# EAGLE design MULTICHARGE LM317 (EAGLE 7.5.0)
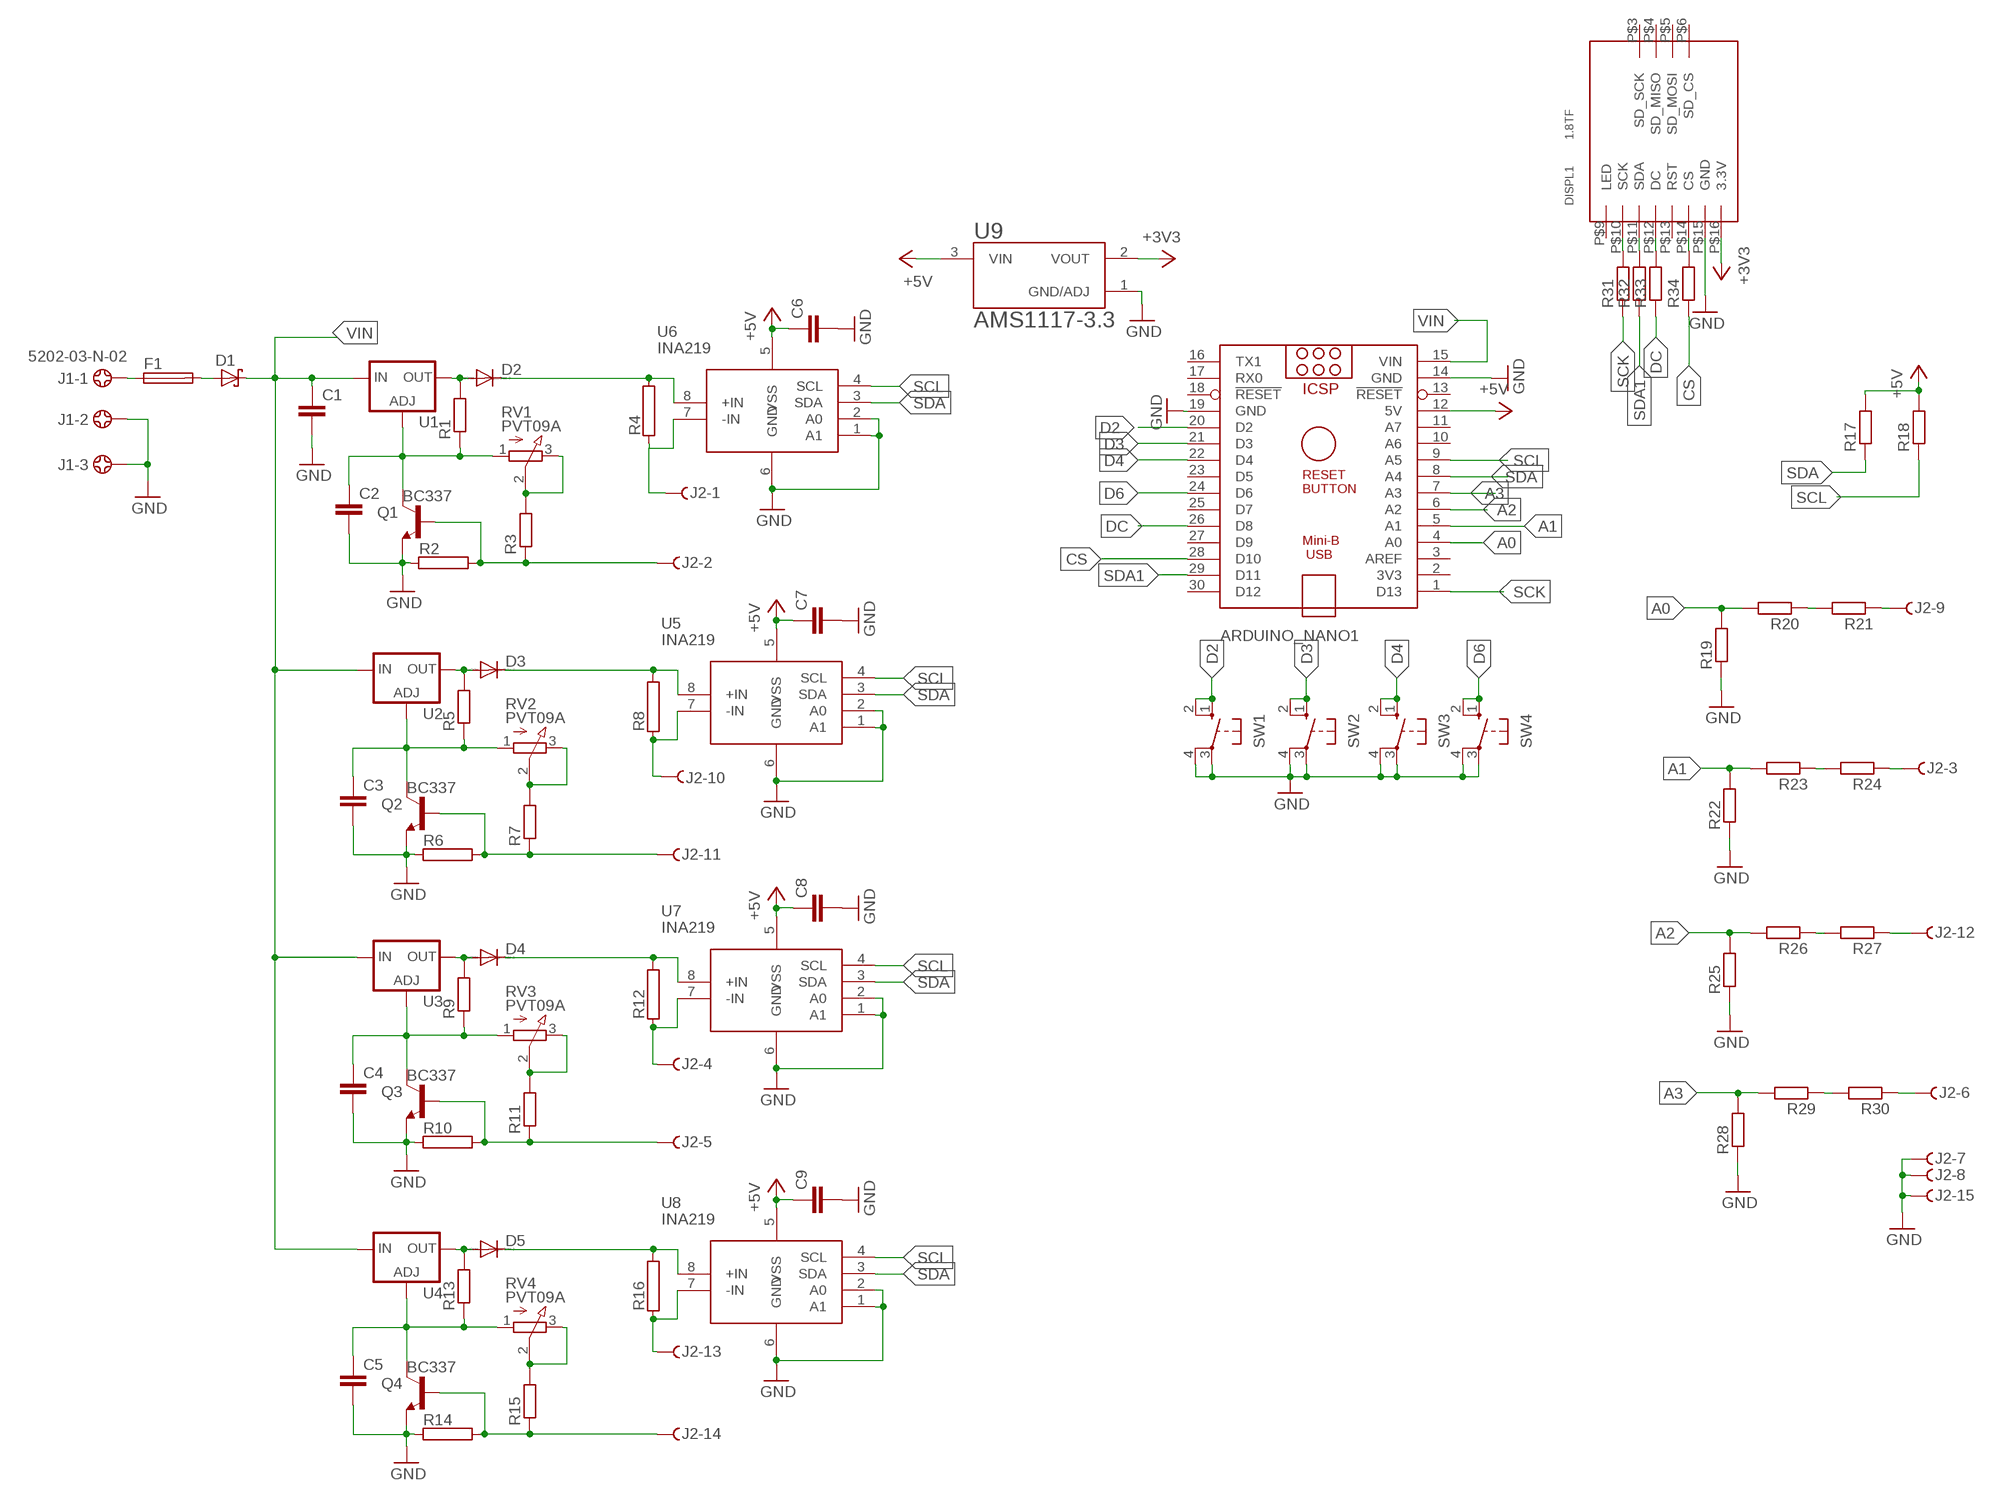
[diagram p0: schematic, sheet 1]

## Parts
ARDUINO_NANO1  ARDUINO_NANO  [ARDUINO_NANO]
C1  C-EUC1206  [C1206]
C2  C-EUC1206  [C1206]
C3  C-EUC1206  [C1206]
C4  C-EUC1206  [C1206]
C5  C-EUC1206  [C1206]
C6  C-EUC0805  [C0805]
C7  C-EUC0805  [C0805]
C8  C-EUC0805  [C0805]
C9  C-EUC1206  [C1206]
D1  MBR1560  [TO220ACS]
D2  CGRM4007-G  [SOD-123_MINI-SMA]
D3  CGRM4007-G  [SOD-123_MINI-SMA]
D4  CGRM4007-G  [SOD-123_MINI-SMA]
D5  CGRM4007-G  [SOD-123_MINI-SMA]
DISPL1  1.8TF  [1.8TFT]
F1  SH22  [SH22]
J1  5202-03-N-02  [5202-03-N-02]
J2  F15.590S  [177-015-212-FEMALE]
Q1  BC337  [TO92]
Q2  BC337  [TO92]
Q3  BC337  [TO92]
Q4  BC337  [TO92]
R1  R-EU_R1206  [R1206]
R2  RAC01  [AC01]
R3  R-EU_R1206  [R1206]
R4  RAC01  [AC01]
R5  R-EU_R1206  [R1206]
R6  RAC01  [AC01]
R7  R-EU_R1206  [R1206]
R8  RAC01  [AC01]
R9  R-EU_R1206  [R1206]
R10  RAC01  [AC01]
R11  R-EU_R1206  [R1206]
R12  RAC01  [AC01]
R13  R-EU_R1206  [R1206]
R14  RAC01  [AC01]
R15  R-EU_R1206  [R1206]
R16  RAC01  [AC01]
R17  R-EU_R1206  [R1206]
R18  R-EU_R1206  [R1206]
R19  R-EU_R1206  [R1206]
R20  R-EU_R1206  [R1206]
R21  R-EU_R1206  [R1206]
R22  R-EU_R1206  [R1206]
R23  R-EU_R1206  [R1206]
R24  R-EU_R1206  [R1206]
R25  R-EU_R1206  [R1206]
R26  R-EU_R1206  [R1206]
R27  R-EU_R1206  [R1206]
R28  R-EU_R1206  [R1206]
R29  R-EU_R1206  [R1206]
R30  R-EU_R1206  [R1206]
R31  R-EU_R1206  [R1206]
R32  R-EU_R1206  [R1206]
R33  R-EU_R1206  [R1206]
R34  R-EU_R1206  [R1206]
RV1  PVT09A  PV09A  [PTV09]
RV2  PVT09A  PV09A  [PTV09]
RV3  PVT09A  PV09A  [PTV09]
RV4  PVT09A  PV09A  [PTV09]
SW1  10-XX  [B3F-10XX]
SW2  10-XX  [B3F-10XX]
SW3  10-XX  [B3F-10XX]
SW4  10-XX  [B3F-10XX]
U1  LM317TS  [317TS]
U2  LM317TS  [317TS]
U3  LM317TS  [317TS]
U4  LM317TS  [317TS]
U5  INA219  [SO08]
U6  INA219  [SO08]
U7  INA219  [SO08]
U8  INA219  [SO08]
U9  AMS1117-3.3  [SOT229P700X180-4N]

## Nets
+3V3: DISPL1.P$16(3.3V) U9.2(VOUT)
+5V: ARDUINO_NANO1.12(5V) C6.1 C7.1 C8.1 C9.1 R17.2 R18.2 U5.5(VSS) U6.5(VSS) U7.5(VSS) U8.5(VSS) U9.3(VIN)
A0: ARDUINO_NANO1.4(A0) R19.2 R20.2
A1: ARDUINO_NANO1.5(A1) R22.2 R23.2
A2: ARDUINO_NANO1.6(A2) R25.2 R26.2
A3: ARDUINO_NANO1.7(A3) R28.2 R29.2
CS: ARDUINO_NANO1.28(D10) R34.1
D2: ARDUINO_NANO1.20(D2) SW1.1(S) SW1.2(S1)
D3: ARDUINO_NANO1.21(D3) SW2.1(S) SW2.2(S1)
D4: ARDUINO_NANO1.22(D4) SW3.1(S) SW3.2(S1)
D6: ARDUINO_NANO1.24(D6) SW4.1(S) SW4.2(S1)
DC: ARDUINO_NANO1.26(D8) R33.1
GND: ARDUINO_NANO1.14(GND) ARDUINO_NANO1.19(GND) C1.2 C2.2 C3.2 C4.2 C5.2 C6.2 C7.2 C8.2 C9.2 DISPL1.P$15(GND) J1.2 J1.3 J2.7 J2.8 J2.15 Q1.1(E) Q2.1(E) Q3.1(E) Q4.1(E) R2.1 R6.1 R10.1 R14.1 R19.1 R22.1 R25.1 R28.1 SW1.3(P) SW1.4(P1) SW2.3(P) SW2.4(P1) SW3.3(P) SW3.4(P1) SW4.3(P) SW4.4(P1) U5.1(A1) U5.2(A0) U5.6(GND) U6.1(A1) U6.2(A0) U6.6(GND) U7.1(A1) U7.2(A0) U7.6(GND) U8.1(A1) U8.2(A0) U8.6(GND) U9.1(GND/ADJ)
N$1: D1.A F1.2
N$2: F1.1 J1.1
N$4: D2.A R1.2 U1.2(OUT)
N$5: C2.1 Q1.3(C) R1.1 RV1.1(A) U1.1(ADJ)
N$6: R3.2 RV1.2(S) RV1.3(E)
N$7: R23.1 R24.2
N$8: J2.2 Q1.2(B) R2.2 R3.1
N$9: D3.A R5.2 U2.2(OUT)
N$10: C3.1 Q2.3(C) R5.1 RV2.1(A) U2.1(ADJ)
N$11: J2.11 Q2.2(B) R6.2 R7.1
N$12: D2.C R4.2 U6.8(+IN)
N$13: J2.1 R4.1 U6.7(-IN)
N$14: R7.2 RV2.2(S) RV2.3(E)
N$15: D3.C R8.2 U5.8(+IN)
N$16: J2.10 R8.1 U5.7(-IN)
N$17: D4.A R9.2 U3.2(OUT)
N$18: C4.1 Q3.3(C) R9.1 RV3.1(A) U3.1(ADJ)
N$19: J2.5 Q3.2(B) R10.2 R11.1
N$20: R11.2 RV3.2(S) RV3.3(E)
N$21: D4.C R12.2 U7.8(+IN)
N$22: J2.4 R12.1 U7.7(-IN)
N$23: D5.A R13.2 U4.2(OUT)
N$24: C5.1 Q4.3(C) R13.1 RV4.1(A) U4.1(ADJ)
N$25: J2.14 Q4.2(B) R14.2 R15.1
N$26: R15.2 RV4.2(S) RV4.3(E)
N$27: D5.C R16.2 U8.8(+IN)
N$28: J2.13 R16.1 U8.7(-IN)
N$29: R20.1 R21.2
N$30: J2.9 R21.1
N$31: J2.3 R24.1
N$32: R26.1 R27.2
N$34: R29.1 R30.2
N$35: J2.12 R27.1
N$37: J2.6 R30.1
N$50: DISPL1.P$10(SCK) R31.2
N$51: DISPL1.P$11(SDA) R32.2
N$52: DISPL1.P$12(DC) R33.2
N$53: DISPL1.P$14(CS) R34.2
SCK: ARDUINO_NANO1.1(D13) R31.1
SCL: ARDUINO_NANO1.9(A5) R18.1 U5.4(SCL) U6.4(SCL) U7.4(SCL) U8.4(SCL)
SDA: ARDUINO_NANO1.8(A4) R17.1 U5.3(SDA) U6.3(SDA) U7.3(SDA) U8.3(SDA)
SDA1: ARDUINO_NANO1.29(D11) R32.1
VIN: ARDUINO_NANO1.15(VIN) C1.1 D1.C U1.3(IN) U2.3(IN) U3.3(IN) U4.3(IN)
Unconnected: ARDUINO_NANO1.2(3V3) ARDUINO_NANO1.3(AREF) ARDUINO_NANO1.10(A6) ARDUINO_NANO1.11(A7) ARDUINO_NANO1.13(!RESET) ARDUINO_NANO1.16(TX1) ARDUINO_NANO1.17(RX0) ARDUINO_NANO1.18(!RESET) ARDUINO_NANO1.23(D5) ARDUINO_NANO1.25(D7) ARDUINO_NANO1.27(D9) ARDUINO_NANO1.30(D12) DISPL1.P$3(SD_SCK) DISPL1.P$4(SD_MISO) DISPL1.P$5(SD_MOSI) DISPL1.P$6(SD_CS) DISPL1.P$9(LED) DISPL1.P$13(RST)

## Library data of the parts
ARDUINO_NANO1 = ArduinoNanoV30:ARDUINO_NANO: Arduino Nano V3.0 Overview: The Arduino Nano is a small, complete, and breadboard-friendly board based on the ATmega328 (Arduino Nano 3.x) or ATmega168 (Arduino Nano 2.x). It has more or less the same functionality of the Arduino Duemilanove, but in a different package. It lacks only a DC power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
C1-C9 = rcl:C-EU: CAPACITOR, European symbol
D1 = diode:MBR1560
D2-D5 = diode:CGRM400*-G: Molded plasitc,JEDEC SOD-123/Mini SMA
DISPL1 = tft_1_8_1_44_oled_0_96:1.8TF
F1 = fuse:SH22: FUSE HOLDER; OC_FARNELL: unknown; OC_NEWARK: unknown
J1 = con-ebyelectro:5202-03-N-02: Barrier Blocks Sreies 5202 Source: http://www.ebyelectro.com/PDF/5202-XX-N-02.pdf; OC_FARNELL: unknown; OC_NEWARK: unknown
J2 = con-subd:F15?S: SUB-D; OC_FARNELL: unknown; OC_NEWARK: unknown
Q1-Q4 = transistor:BC337: NPN TRANSISTOR
R1 R3 R5 R7 R9 R11 R13 R15 R17-R34 = rcl:R-EU_: RESISTOR, European symbol
R2 R4 R6 R8 R10 R12 R14 R16 = resistor-power:R: Power Resitor; OC_FARNELL: unknown; OC_NEWARK: unknown
RV1-RV4 = pot:PV09A
SW1-SW4 = switch-omron:10-XX: OMRON SWITCH; MPN: B3F-1000; OC_FARNELL: 176432; OC_NEWARK: 36M3542
U1-U4 = v-reg:LM317TS: VOLTAGE REGULATOR
U5-U8 = burr-brown:INA219: Bidirectional Current/Power Monitor With I2C Interface
U9 = AMS1117-3.3:AMS1117-3.3: Check availability; AVAILABILITY: Not in stock; CHECK_PRICES: https://www.snapeda.com/parts/AMS1117-3.3/Advanced+Monolithic+Systems/view-part/?ref=eda; DESCRIPTION: Sot223/Pkg 1-Amp 3.3-Volt Low Drop Out Voltage Regulatator; MF: Advanced Monolithic Systems; MP: AMS1117-3.3; PACKAGE: SOT-223 Seeed Technology; PRICE: None; SNAPEDA_LINK: https://www.snapeda.com/parts/AMS1117-3.3/Advanced+Monolithic+Systems/view-part/?ref=snap

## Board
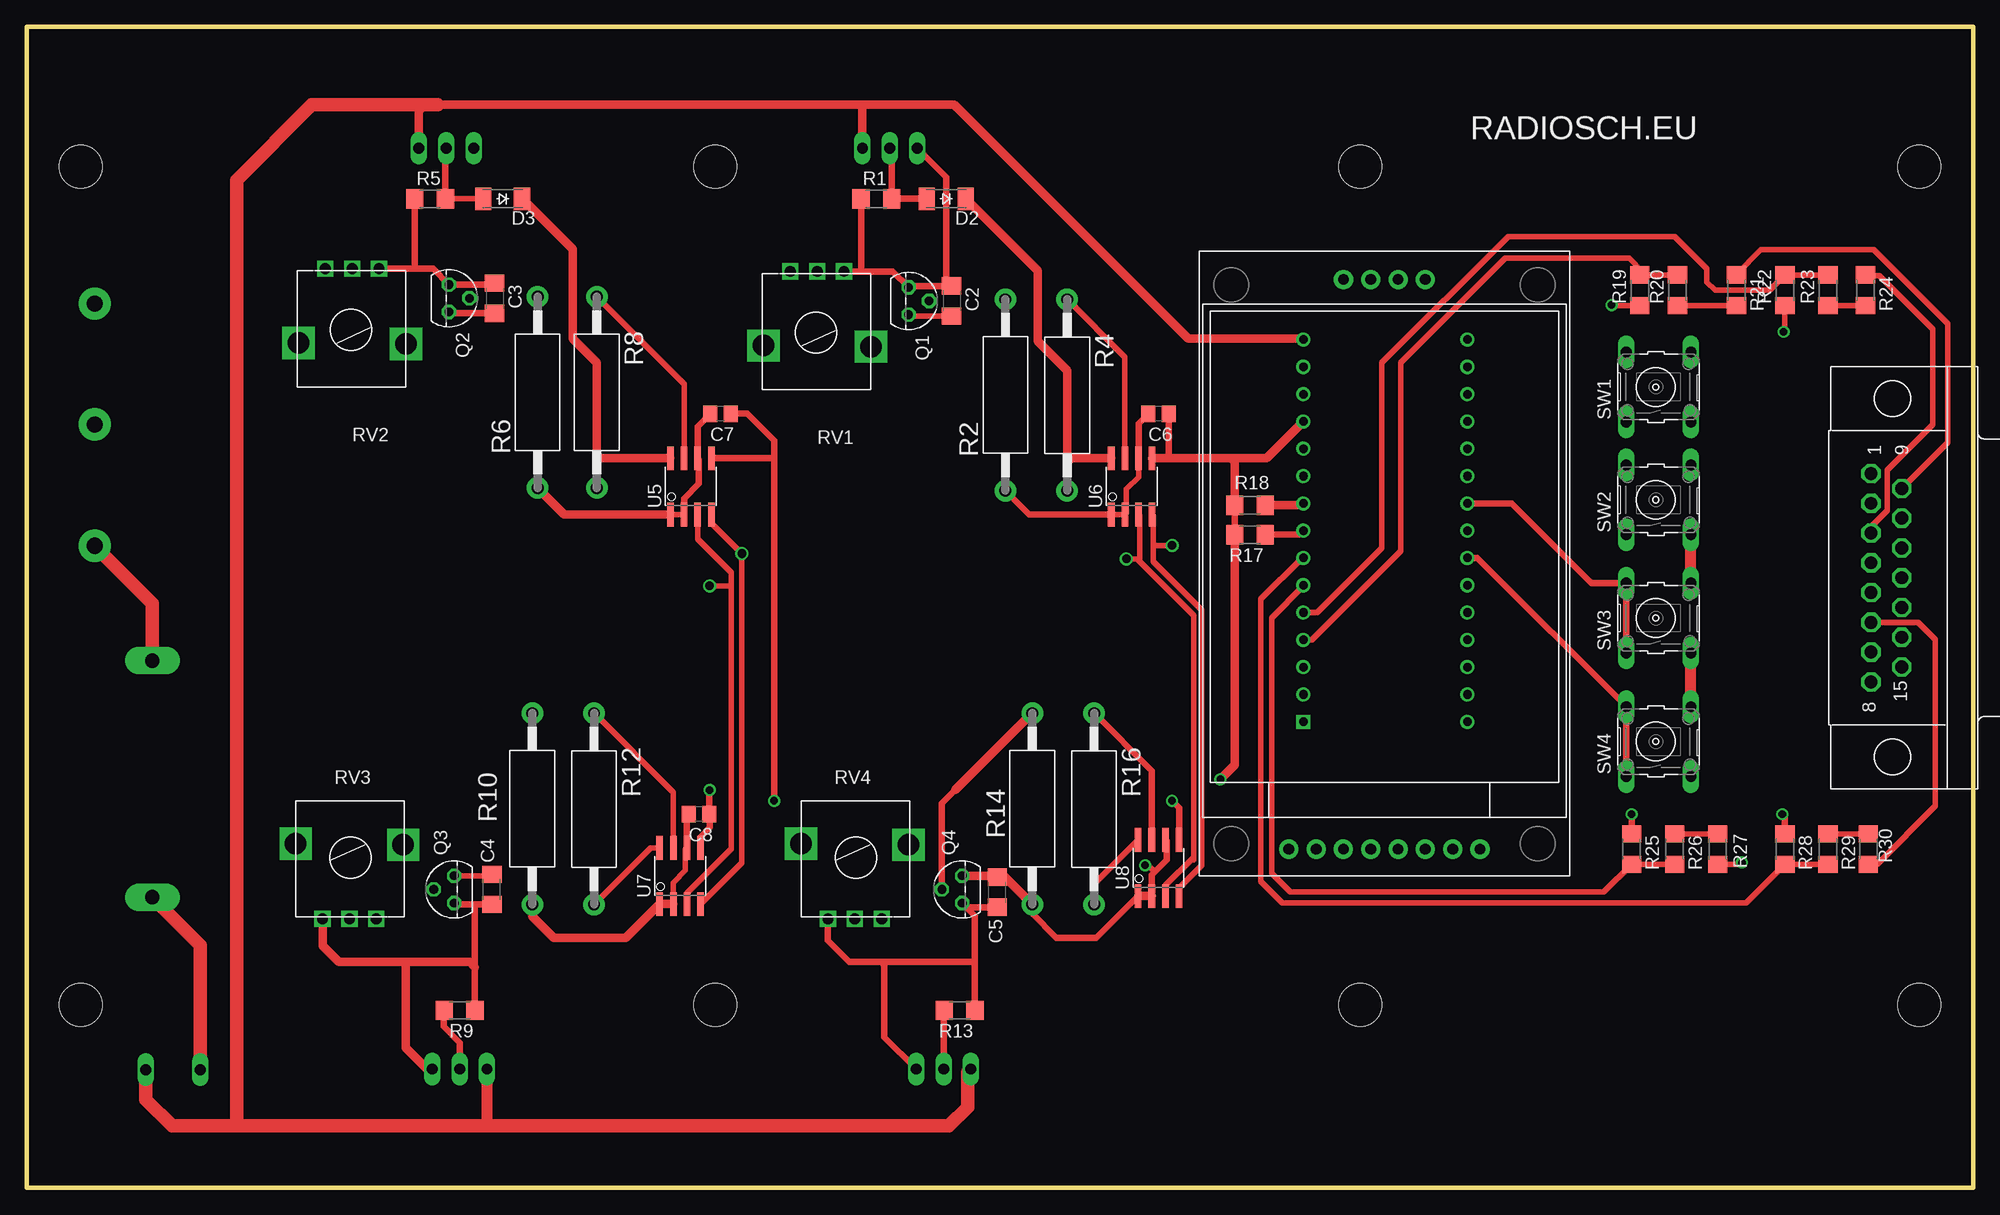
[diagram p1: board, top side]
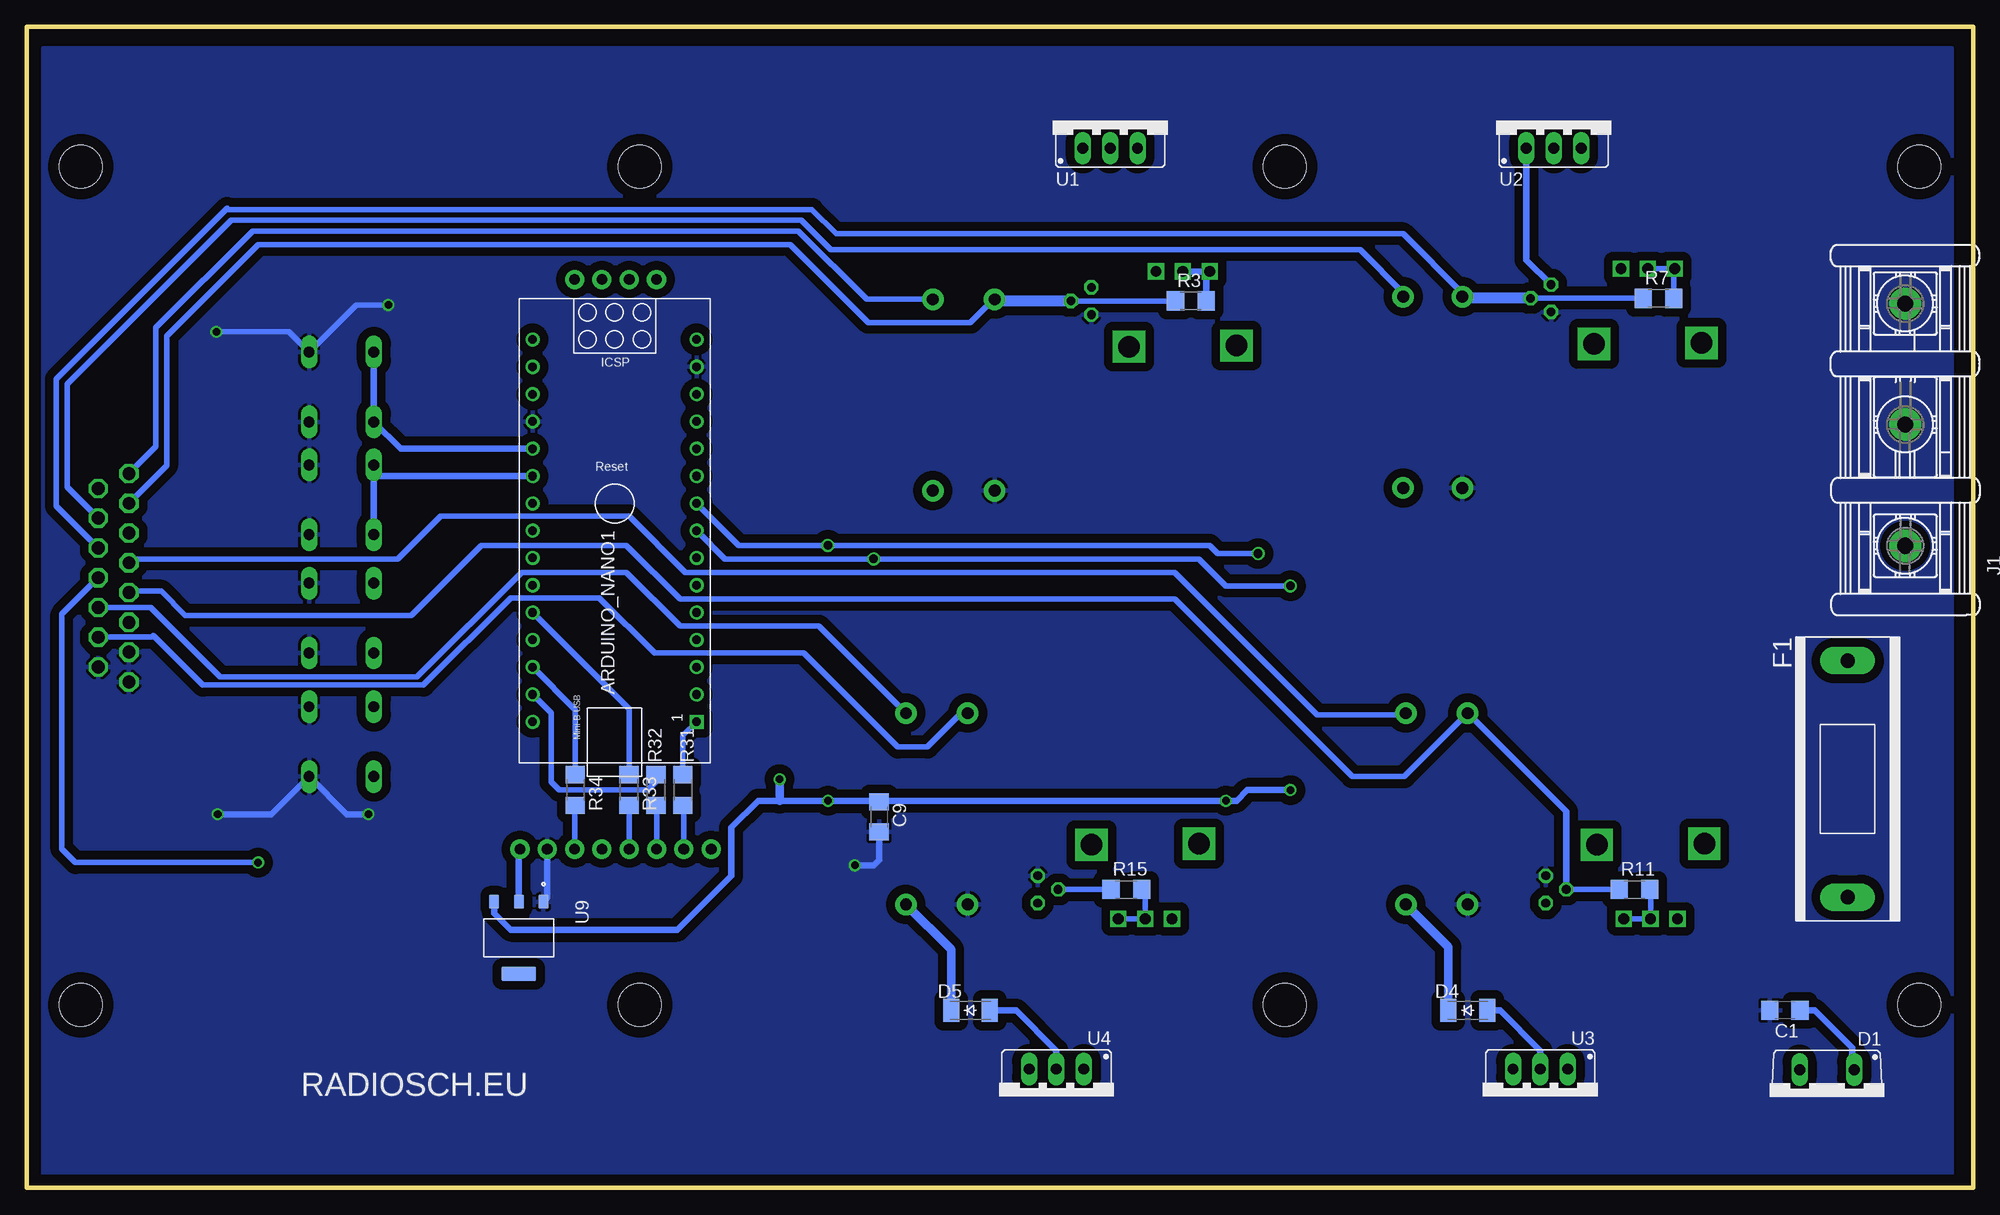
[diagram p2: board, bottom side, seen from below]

Size 181 x 108 mm. Coordinates in mm from the lower left corner, seen from the top.
Outline: 0,0 181,0 181,108 0,108 0,0
Copper layers (1*16): Top 0.035mm / dielectric 1.5mm / Bottom 0.035mm
Design rules "default": minimum track width 10mil, minimum drill 24mil, track to track 8mil, track to pad 8mil, pad to pad 8mil, via to via 8mil, smd to smd 8mil, copper to edge 40mil, drill to drill 8mil, minimum pad ring 10mil, minimum via ring 8mil, stop-mask expansion 4mil, vias tented up to drill 0mil, thermal gap 10mil
Holes 4 mm at 5,95 5,17 176,17 176,95 64,17 124,17 64,95 124,95

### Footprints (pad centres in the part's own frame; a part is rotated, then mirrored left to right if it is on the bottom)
ARDUINO_NANO = drill 0.8 square: 1 -20.32,-7.62 | drill 0.8: 2 -17.78,-7.62; 3 -15.24,-7.62; 4 -12.7,-7.62; 5 -10.16,-7.62; 6 -7.62,-7.62; 7 -5.08,-7.62; 8 -2.54,-7.62; 9 0,-7.62; 10 2.54,-7.62; 11 5.08,-7.62; 12 7.62,-7.62; 13 10.16,-7.62; 14 12.7,-7.62; 15 15.24,-7.62; 16 15.24,7.62; 17 12.7,7.62; 18 10.16,7.62; 19 7.62,7.62; 20 5.08,7.62; 21 2.54,7.62; 22 0,7.62; 23 -2.54,7.62; 24 -5.08,7.62; 25 -7.62,7.62; 26 -10.16,7.62; 27 -12.7,7.62; 28 -15.24,7.62; 29 -17.78,7.62; 30 -20.32,7.62
C1206 = smd 1.6 x 1.8: 1 -1.4,0; 2 1.4,0
C0805 = smd 1.3 x 1.5: 1 -0.95,0; 2 0.95,0
TO220ACS = drill 1.016 long: A 2.54,-2.54; C -2.54,-2.54
SOD-123_MINI-SMA = smd 1.5 x 2.1: A 1.8,0; C -1.8,0
1.8TFT = drill 1 pad 1.778: P$3 55.5,21.05; P$4 55.5,18.52; P$5 55.5,15.98; P$6 55.5,13.44; P$9 2.5,26.14; P$10 2.5,23.6; P$11 2.5,21.06; P$12 2.5,18.52; P$13 2.5,15.98; P$14 2.5,13.44; P$15 2.5,10.9; P$16 2.5,8.36
SH22 = drill 1.321 pad 2.54 long: 1 -10.998,0; 2 10.998,0
5202-03-N-02 = drill 1.5 pad 3: 1 -9.29,0; 2 2,0; 3 13.25,0
177-015-212-FEMALE = drill 1.194 pad 1.524 octagon: 1 -9.69,-1.99; 2 -6.921,-1.99; 3 -4.153,-1.99; 4 -1.384,-1.99; 5 1.384,-1.99; 6 4.153,-1.99; 7 6.921,-1.99; 8 9.69,-1.99; 9 -8.306,0.854; 10 -5.537,0.854; 11 -2.769,0.854; 12 0,0.854; 13 2.769,0.854; 14 5.537,0.854; 15 8.306,0.854
TO92 = drill 0.813 octagon: 1 1.27,0; 2 0,1.905; 3 -1.27,0
R1206 = smd 1.6 x 1.803: 1 -1.422,0; 2 1.422,0
AC01 = drill 1.1 pad 2: 1 -8.9,0; 2 8.9,0
PTV09 = drill 1 square: 1 -2.5,0; 2 0,0; 3 2.5,0 | drill 2 square: P$4 -5,7; P$5 5,6.9
B3F-10XX = drill 1.016 long: 1 -3.251,2.761; 2 3.251,2.761; 3 -3.251,-3.261; 4 3.251,-3.261
317TS = drill 1.016 long: 1 -2.54,-2.54; 2 0,-2.54; 3 2.54,-2.54
SO08 = smd 0.61 x 2.21: 1 -1.905,-2.616; 2 -0.635,-2.616; 3 0.635,-2.616; 4 1.905,-2.616; 5 1.905,2.616; 6 0.635,2.616; 7 -0.635,2.616; 8 -1.905,2.616
SOT229P700X180-4N = smd 1.31 x 0.93: 1 -3.345,2.29; 2 -3.345,0; 3 -3.345,-2.29 | smd 1.31 x 3.24: 4 3.345,0

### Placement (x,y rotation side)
ARDUINO_NANO1  126.34,63.67 90 bottom
C1  17.5,16.5 180 bottom
C2  86,82.5 270 top
C3  43.5,82.75 270 top
C4  43.25,27.75 90 top
C5  90.25,27.5 90 top
C6  105.25,72 180 top
C7  64.5,72 180 top
C8  62.5,34.75 180 top
C9  101.75,34.5 270 bottom
D1  13.6,8.44 180 bottom
D2  85.5,92 180 top
D3  44.25,92 180 top
D4  47,16.5 0 bottom
D5  93.25,16.5 0 bottom
DISPL1  143.5,29 90 top
F1  11.67,38.03 270 bottom
J1  6.32,69.01 90 bottom
J2  173.5,56.75 270 top
Q1  82,82.5 270 top
Q2  39.25,82.75 270 top
Q3  39.75,27.75 90 top
Q4  87,27.75 90 top
R1  79,92 0 top
R2  91,73.75 90 top
R3  72.75,82.5 0 bottom
R4  96.75,73.75 270 top
R5  37.5,92 0 top
R6  47.5,74 90 top
R7  29.25,82.75 0 bottom
R8  53,74 270 top
R9  40.25,16.5 180 top
R10  47,35.25 90 top
R11  31.5,27.75 0 bottom
R12  52.75,35.25 270 top
R13  86.75,16.5 180 top
R14  93.5,35.25 90 top
R15  78.75,27.75 0 bottom
R16  99.25,35.25 270 top
R17  113.75,60.75 180 top
R18  113.75,63.5 180 top
R19  150,83.5 90 top
R20  153.5,83.5 90 top
R21  159,83.5 270 top
R22  163.5,83.5 90 top
R23  167.5,83.5 90 top
R24  171,83.5 270 top
R25  149.25,31.5 270 top
R26  153.25,31.5 270 top
R27  157.25,31.5 90 top
R28  163.5,31.5 270 top
R29  167.5,31.5 270 top
R30  171.25,31.5 90 top
R31  120,37 270 bottom
R32  122.5,37 270 bottom
R33  125,37 270 bottom
R34  130,37 270 bottom
RV1  73.5,85.25 180 top
RV2  30.25,85.5 180 top
RV3  30,25 0 top
RV4  77,25 0 top
SW1  151.5,74.5 90 top
SW2  151.5,64 90 top
SW3  151.5,53 90 top
SW4  151.5,41.5 90 top
U1  80.25,99.25 0 bottom
U2  39,99.25 0 bottom
U3  40.25,8.5 180 bottom
U4  85.25,8.5 180 bottom
U5  61.75,65.25 0 top
U6  102.75,65.25 0 top
U7  60.75,29 0 top
U8  105.25,29.75 0 top
U9  135.25,23.25 270 bottom

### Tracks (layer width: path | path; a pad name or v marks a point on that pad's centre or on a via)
+3V3
  Bottom 0.61: U9.2 135.25,31.39 DISPL1.P$16
+5V  (via drill 0.7)
  Top 0.61: U8.5 107.16,35.34 v106.5,36 | R18.2 R17.2 | U7.5 62.66,32.66 63.5,33.5 63.5,34.7 C8.1 63.45,36.95 v63.5,37 | 69.5,68 69.5,69.5 67,72 C7.1 | 69.5,68 v69.5,36 | U5.5 69.37,67.87 69.5,68 | C6.1 106.2,67.94 106.12,67.87
  Top 0.813: 104.66,67.84 U6.5 106.12,67.87 112,67.87 | 112,67.87 115.3,67.87 ARDUINO_NANO1.12 | R18.2 112.33,67.54 112,67.87 | R17.2 112.33,39.33 v111,38
  Bottom 0.61: U9.3 137.54,25.54 136,24 120.5,24 115.5,29 115.5,33.5 113,36 111,36 v106.5,36 101.85,36 C9.1 101.65,36 v69.5,36 68.5,36 67.5,37 v63.5,37
  Bottom 0.813: v111,38 111,36
A0
  Top 0.5: 150.25,85.25 149,86.5 137.5,86.5 127.75,76.75 127.75,59.25 119.47,50.97 ARDUINO_NANO1.4 | 150.25,85.25 150.58,84.92 R20.2 | R19.2 150,85 150.25,85.25
A1
  Top 0.5: R23.2 R22.2 162.08,83.5 157,83.5 156.25,84.25 156.25,85.5 153.25,88.5 137.75,88.5 126,76.75 126,59.5 120.01,53.51 ARDUINO_NANO1.5
A2
  Top 0.5: ARDUINO_NANO1.6 118.72,55.97 115.75,53 115.75,29.25 117.5,27.5 146.67,27.5 R25.2 R26.2
A3
  Top 0.5: ARDUINO_NANO1.7 118.59,58.59 114.75,54.75 114.75,28.5 116.75,26.5 159.92,26.5 R28.2 R29.2
CS
  Bottom 0.5: R34.1 130,44.47 ARDUINO_NANO1.28
D2
  Bottom 0.61: SW1.2 SW1.1 146.24,68.75 ARDUINO_NANO1.20
D3
  Bottom 0.61: SW2.1 148.74,66.75 | 148.74,66.75 SW2.2 | ARDUINO_NANO1.21 148.2,66.21 148.74,66.75
D4
  Top 0.61: SW3.1 SW3.2 145.5,56.25 138.08,63.67 ARDUINO_NANO1.22
D6
  Top 0.61: ARDUINO_NANO1.24 134.9,58.59 SW4.2 SW4.1
DC
  Bottom 0.5: R33.1 125,44.55 ARDUINO_NANO1.26
GND  (via drill 0.7)
  Top 0.5: U5.2 U5.1 | U7.2 60.12,28.36 61.25,29.5 61.25,31.48 U7.6 | Q3.1 43.12,29.02 C4.2 | 47,25.25 R10.1 | R19.1 147.42,82.08 v147.38,82.12 | R22.1 163.5,79.75 v163.38,79.62 | U6.6 103.39,66.14 102.25,65 102.25,62.77 U6.2 U6.1 | C2.2 82.13,81.1 Q1.1
  Top 0.61: R14.1 93.5,25.5 95.75,23.25 99.46,23.25 U8.1 | U8.2 104.61,29.11 104.88,29.38 | 104.88,29.38 106,30.5 106,32.25 U8.6 | C5.2 90.25,29.02 | v104,30 104.25,30 104.88,29.38 | C3.2 39.38,81.35 Q2.1 | U7.6 61.38,34.59 C8.2 | U5.2 61.12,64.11 62.5,65.5 62.5,67.75 U5.6 62.38,70.83 C7.2 | R25.1 v149.25,34.75 | R28.1 163.5,34.5 v163.25,34.75 | U6.1 93.22,62.63 R2.1 | U6.6 103.39,71.08 C6.2
  Top 0.813: 47,25.25 49,23.25 55.71,23.25 U7.1 U7.2 | Q4.1 90.25,29.02 90.83,29.02 R14.1 | U8.1 U8.2 | U5.1 49.97,62.63 R6.1
  Top 1.016: SW4.4 SW3.3 | SW3.4 SW2.3
  Bottom 0.5: v147.38,82.12 150.39,82.12 SW1.4 156.63,79.62 v163.38,79.62
  Bottom 0.61: DISPL1.P$15 132.6,26.95 U9.1 | C9.2 101.75,30.5 102.25,30 v104,30 | v149.25,34.75 151.26,34.75 SW4.3 158.26,34.75 v163.25,34.75
  Bottom 0.813: 46.87,26.48 R10.1
  pour Bottom (isolate 0.813): 2,106 179.5,106 179.5,1 2,1
N$1
  Top 1.27: D1.A 16.14,22.56 F1.2
N$2
  Top 1.27: F1.1 11.67,54.37 J1.1
N$4
  Top 0.61: D2.A R1.2 80.42,96.54 U1.2
N$5
  Top 0.61: RV1.1 77.5,85.25 | 77.5,85.25 80.52,85.25 Q1.3 82.13,83.9 C2.1 85.5,84.4 85.5,94 U1.1 | R1.1 77.58,85.33 77.5,85.25
N$6
  Bottom 0.61: R3.2 71.33,84.92 RV1.3 RV1.2
N$7
  Top 0.5: R23.1 R24.2
N$8
  Bottom 0.5: R2.2 91.1,82.65 93.25,80.5 102.75,80.5 110,87.75 159.5,87.75 168,79.25 168,67.18 J2.2 | R3.1 Q1.2
  Bottom 1.016: Q1.2 90.85,82.5 R2.2
N$9
  Top 0.5: R5.2 D3.A
  Top 0.61: R5.2 38.92,96.88 U2.2
N$10
  Top 0.61: RV2.1 36,85.5 | 36,85.5 37.77,85.5 Q2.3 39.98,84.02 40,84 43.35,84 C3.1 | R5.1 36.08,85.58 36,85.5
  Bottom 0.61: U2.1 41.54,86.31 Q2.3
N$11
  Bottom 0.5: R6.2 47.5,83.25 53,88.75 105.75,88.75 108,91 162.25,91 162.38,91.12 178.25,75.25 178.25,63.41 J2.11 | R7.1 Q2.2
  Bottom 1.016: Q2.2 47.35,82.75 R6.2
N$12
  Top 0.813: D2.C 94,85.3 94,78.75 96.75,76 96.75,67.5 | R4.2 96.75,67.5 | U6.8 97.12,67.87 96.75,67.5
N$13
  Top 0.5: U6.7 102.11,77.28 R4.1
  Bottom 0.5: J2.1 169,68.95 169,80 160,89 109.25,89 102.9,82.65 R4.1
N$14
  Bottom 0.5: R7.2 27.83,85.42 RV2.3 RV2.2
N$15
  Top 0.813: R8.2 53,67.75 | 53,67.75 53,76.75 50.75,79 50.75,87.3 D3.C | U5.8 53.12,67.87 53,67.75
N$16
  Top 0.5: U5.7 61.12,74.78 R8.1
  Bottom 0.5: R8.1 53,83.25 57,87.25 106.25,87.25 109,90 162,90 177.25,74.75 177.25,65.18 J2.10
N$17
  Top 0.61: 38.75,16.42 38.75,15 40.25,13.5 U3.2
  Top 0.813: 38.75,16.42 R9.2
  Bottom 0.61: D4.A 44,16.5 40.25,12.75 U3.2
N$18
  Top 0.61: C4.1 41.75,26.35 | 41.75,26.35 39.88,26.35 Q3.3 | R9.1 41.67,20.5 41.67,26.27 41.75,26.35
  Top 0.813: RV3.1 27.5,22.5 29,21 35,21 | 35,21 41.17,21 41.67,20.5 | U3.1 37.21,11.04 35.25,13 35.25,20.75 35,21
N$19
  Bottom 0.5: Q3.2 R11.1 | J2.5 171.38,55.5 168.5,55.5 166.25,53.25 145.25,53.25 138.75,59.75 125.25,59.75 120.25,54.75 74.25,54.75 57.75,38.25 52.9,38.25 R10.2
  Bottom 0.61: Q3.2 37.84,34.99 R10.2
  Bottom 0.813: R10.2 47.35,44.15
N$20
  Bottom 0.5: R11.2 30,27.67 RV3.2 RV3.3
N$21
  Top 0.5: U7.8 58.02,31.62 R12.2
  Bottom 0.813: D4.C 48.8,22.4 R12.2
N$22
  Top 0.5: U7.7 60.12,36.78 R12.1
  Bottom 0.5: J2.4 171.14,58.5 146.5,58.5 142.5,62.5 125,62.5 119.75,57.25 74.25,57.25 61,44 52.9,44 R12.1
N$23
  Top 0.61: U4.2 85.25,16.42 R13.2
  Bottom 0.61: D5.A 89,16.5 85.25,12.75 U4.2
N$24
  Top 0.61: R13.1 88.17,21 | 88.17,21 88.17,25.31 Q4.3 87.38,26.1 C5.1 | RV4.1 74.5,23 76.5,21 79.5,21 | 79.5,21 88.17,21 | U4.1 79.75,14 79.75,20.75 79.5,21
N$25
  Top 0.61: Q4.2 85.09,35.74 86.34,36.99
  Top 0.813: 86.34,36.99 R14.2
  Bottom 0.5: Q4.2 R15.1 | R14.2 94.1,44.15 97.25,41 100,41 108.75,49.75 122.62,49.75 127.75,54.88 136,54.88 144.12,46.75 164.62,46.75 168.81,50.94 169.09,51.21 | 169.09,51.21 169.25,51.38 | J2.14 169.09,51.21
N$26
  Bottom 0.5: R15.2 77,27.42 RV4.2 RV4.3
N$27
  Top 0.5: R16.2 99.25,28.27 U8.8
  Bottom 0.813: D5.C 95.05,22.15 R16.2
N$28
  Top 0.61: U8.7 104.61,38.78 R16.1
  Bottom 0.5: J2.13 169.48,53.98 163,47.5 144.75,47.5 135,57.25 125.25,57.25 120.25,52.25 107.35,52.25 R16.1
N$29
  Top 0.5: R20.1 R21.2
N$30
  Top 0.5: J2.9 178.62,69.33 178.62,80.38 171.75,87.25 161.25,87.25 159,85 R21.1
N$31
  Top 0.5: J2.3 171.51,61.51 173,63 173,66.75 177.25,71 177.25,79.88 172.25,84.88 171.05,84.88 R24.1
N$32
  Top 0.5: R27.2 R26.1
N$34
  Top 0.5: R29.1 R30.2
N$35  (via drill 0.7)
  Top 0.5: R27.1 159.33,30.08 v159.5,30.25
  Bottom 0.5: v159.5,30.25 176.5,30.25 177.75,31.5 177.75,53.35 J2.12
N$37
  Top 0.5: R30.1 172.08,30.08 177.5,35.5 177.5,51 175.9,52.6 J2.6
N$50
  Bottom 0.5: DISPL1.P$10 119.9,35.48 R31.2
N$51
  Bottom 0.5: DISPL1.P$11 122.44,35.52 R32.2
N$52
  Bottom 0.5: DISPL1.P$12 124.98,35.56 R33.2
N$53
  Bottom 0.5: DISPL1.P$14 130.06,35.52 R34.2
SCK
  Bottom 0.5: R31.1 120,42.07 ARDUINO_NANO1.1
SCL  (via drill 0.8)
  Top 0.5: U5.4 63.66,61.84 v66.5,59 66.5,30.23 U7.4 | U8.4 107.16,27.91 109.25,30 109.25,53.75 104.75,58.25 104.75,59.75 | 104.75,59.75 104.75,62.54 U6.4 | v106.5,59.75 104.75,59.75
  Top 0.813: R18.1 118.55,63.5 ARDUINO_NANO1.9
  Bottom 0.5: v66.5,59 70.25,59 71,59.75 v106.5,59.75 114.8,59.75 ARDUINO_NANO1.9
SDA  (via drill 0.8)
  Top 0.5: U5.3 62.38,60.37 65.5,57.25 65.5,56 | U7.3 61.38,27.39 65.5,31.5 65.5,56 | U8.3 105.89,28.14 108.5,30.75 | 108.5,30.5 108.5,30.75 | 108.5,30.75 108.5,53.25 103.5,58.25 | 103.5,58.25 103.5,62.52 U6.3 | 65.5,56 v63.5,56 | v102.25,58.5 103.25,58.5 103.5,58.25
  Top 0.61: R17.1 118.34,60.75 ARDUINO_NANO1.8
  Bottom 0.5: v63.5,56 69.5,56 72,58.5 v102.25,58.5 116.09,58.5 ARDUINO_NANO1.8
SDA1
  Bottom 0.5: R32.1 122.5,37.75 123.25,37 131.5,37 132.25,37.75 132.25,44.18 ARDUINO_NANO1.29
VIN
  Top 0.813: ARDUINO_NANO1.15 118.63,79 108,79 86.25,100.75 77.75,100.75 | 77.75,100.75 38.21,100.75 | U2.3 36.46,100.21 37,100.75 | U1.3 77.71,100.71 77.75,100.75
  Top 1.016: U3.3 42.79,6.21 43.25,5.75
  Top 1.27: 38.21,100.75 37,100.75 26.5,100.75 19.5,93.75 19.5,5.75 | D1.C 11.06,8.19 13.5,5.75 19.5,5.75 | 19.5,5.75 43.25,5.75 85.75,5.75 87.5,7.5 87.5,10.75 U4.3
  Bottom 0.61: C1.1 14.75,16.5 11.25,13 11.25,11.17 D1.C

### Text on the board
tPlace: RADIOSCH.EU
bPlace: RADIOSCH.EU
